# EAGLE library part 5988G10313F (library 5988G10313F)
LED, Red, Green, Blue, SMD, 110 , Square, R 20mA, G 20mA, B 20mA Source: Datasheet
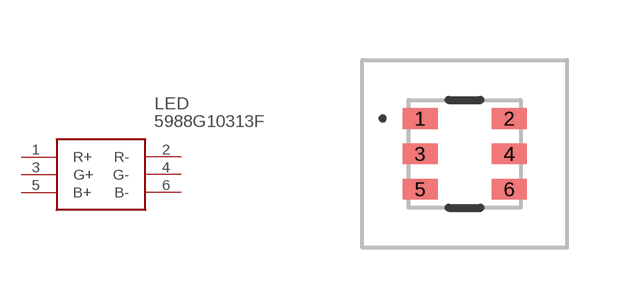
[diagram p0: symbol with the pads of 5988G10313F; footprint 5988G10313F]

Designator prefix LED

## 5988G10313F (Description: LED, Red, Green, Blue, SMD, 110 , Square, R 20mA, G 20mA, B 20mA; Height: 2.577mm; Manufacturer_Name: Dialight; Manufacturer_Part_Number: 5988G10313F; Mouser_Part_Number: 645-5988G10313F; Mouser_Price-Stock: https://www.mouser.co.uk/ProductDetail/Dialight/5988G10313F?qs=zW32dvEIR3sBNt7cJtOHTg%3D%3D)  [5988G10313F]
1  R+
2  R-
3  G+
4  G-
5  B+
6  B-

## Footprint 5988G10313F (pad centres in mm)
5988G10313F-1
smd 0.88 x 0.52: 1 -1.115,0.885; 2 1.115,0.885; 3 -1.115,0; 4 1.115,0; 5 -1.115,-0.885; 6 1.115,-0.885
